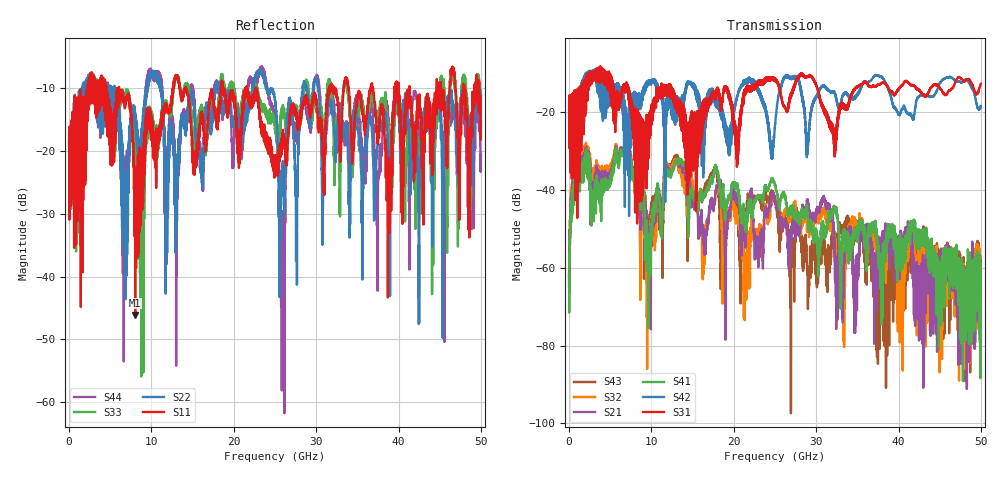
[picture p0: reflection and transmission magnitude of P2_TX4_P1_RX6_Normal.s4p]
!Keysight Technologies,N5225B,MY57041031,A.13.20.10
!Date: Friday, May 31, 2019 11:23:26
!Correction: S11(Full 4 Port(1,2,3,4))
!S12(Full 4 Port(1,2,3,4))
!S13(Full 4 Port(1,2,3,4))
!S14(Full 4 Port(1,2,3,4))
!S21(Full 4 Port(1,2,3,4))
!S22(Full 4 Port(1,2,3,4))
!S23(Full 4 Port(1,2,3,4))
!S24(Full 4 Port(1,2,3,4))
!S31(Full 4 Port(1,2,3,4))
!S32(Full 4 Port(1,2,3,4))
!S33(Full 4 Port(1,2,3,4))
!S34(Full 4 Port(1,2,3,4))
!S41(Full 4 Port(1,2,3,4))
!S42(Full 4 Port(1,2,3,4))
!S43(Full 4 Port(1,2,3,4))
!S44(Full 4 Port(1,2,3,4))
!S4P File: Measurements: <S11,S12,S13,S14>,
!<S21,S22,S23,S24>,
!<S31,S32,S33,S34>,
!<S41,S42,S43,S44>:
# Hz S  dB  R 50.0
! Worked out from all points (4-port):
!   5000 points, 10 MHz to 50 GHz, reference 50 ohm
!   strongest paths, dB at 10 MHz, 12.51 GHz, 25.01 GHz, 37.51 GHz, 50 GHz:
!     S31: -19.3, -14.3, -11.4, -12.8, -12.6
!     S42: -19.4, -15.6, -23.0, -10.6, -18.3
!     S41: -61.8, -35.4, -38.7, -56.7, -68.5
!     S21: -65.1, -35.3, -42.4, -61.8, -73.3
!     S32: -61.5, -33.9, -41.9, -60.0, -74.2
!     S43: -61.3, -32.8, -43.1, -60.6, -63.3
!   lowest |S11| = -46.1 dB at 8.03 GHz (marker M1), VSWR 1.01, Z = 50.3 - j0.417 ohm
!   |S11| at or under -10 dB: 6.073 GHz to 12.61 GHz (6.542 GHz wide, 70 % of centre); 14.2 GHz to 18.43 GHz (4.229 GHz wide, 25.9 % of centre); 22.71 GHz to 31.61 GHz (8.893 GHz wide, 32.7 % of centre)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
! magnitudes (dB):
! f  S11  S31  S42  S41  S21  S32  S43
! 10 MHz  -18.9  -19.3  -19.4  -61.8  -65.1  -61.5  -61.3
! 1.87 GHz  -19.7  -19.7  -12.1  -31.7  -30.4  -28.7  -29.9
! 8.03 GHz  -46.1  -23.4  -19.2  -39.1  -38.9  -42.0  -41.6
! 23.47 GHz  -17.3  -12.7  -17.6  -42.9  -53.3  -54.0  -44.9
! 25.9 GHz  -17.9  -17.3  -12.1  -41.5  -48.3  -48.4  -48.7
! 30.05 GHz  -12.3  -13.2  -16.0  -50.6  -44.9  -46.3  -62.2
! 50 GHz  -15.3  -12.6  -18.3  -68.5  -73.3  -74.2  -63.3
